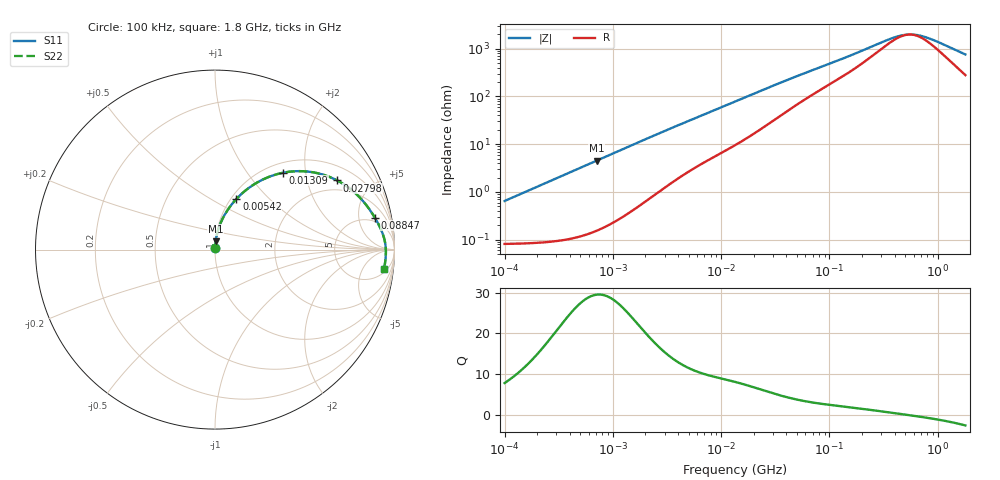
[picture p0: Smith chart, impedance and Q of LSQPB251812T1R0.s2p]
! LSQPB251812T1R0  S-PARAMETER MODEL  ( General Type )
! Model Generated by TAIYO YUDEN Corporation (http://www.ty-top.com)
! Version 3.0
! TAIYO YUDEN Control No. 110926NF18SB-HKC
! Copyright(c) 2007 TAIYO YUDEN CO.,LTD. All Rights Reserved.
! Product Description (link to TY-COMPAS)
! https://ds.yuden.co.jp/TYCOMPAS/or/detail?pn=LSQPB251812T1R0M&u=M
! Products Name : Inductors
! Characteristics :
!  Inductance : 1.0 uH , SRF(min) : 130 MHz , DC Resistance(max) : 0.104 Ohm
!  Rated Current : Saturation :1600 mA , Temp Rise : 1000 mA (40 degC)
!  Case Size : 2.5 x 1.8 / 0.098 x 0.071 [mm/inch] , Thickness : 1.2 / 0.048 [mm/inch]
!  (Conditions: Temperature = 25 degC , DC Bias Current/Voltage = 0A / 0V)
! External Node Assignments :
!  1  o---GGG---o  2
! GND o---------o GND
! Frequency Range : 0.1MHz  -  1800MHz  [ 402 STEP ]
# MHz S RI R 50
! Freq[MHz].  S11 Real  S11 Imag  S21 Real  S21 Imag  S12 Real  S12 Imag  S22 Real  S22 Imag
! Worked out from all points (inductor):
!   401 points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, 100 kHz to 1.8 GHz, reference 50 ohm
!   read as one part in series: L = 1.02 uH near 105 kHz
!   highest Q = 29.5 at 709.7 kHz (marker M1), where L = 1.02 uH
!   self-resonance near 546.1 MHz
!   S11 on the Smith chart (normalised r, x): 100 kHz: 1.00, +0.01; 5.42 MHz: 1.06, +0.66; 13.09 MHz: 1.18, +1.51; 27.98 MHz: 1.55, +3.08; 88.47 MHz: 4.01, +8.15; 1.8 GHz: 7, -14
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0.1  0.000855 0.0064  0.9991 -0.0064  0.9991 -0.0064  0.000855 0.0064
0.516129  0.00228 0.0329  0.9977 -0.0329  0.9977 -0.0329  0.00228 0.0329
0.709667  0.00359 0.0452  0.9964 -0.0452  0.9964 -0.0452  0.00359 0.0452
1.443982  0.0121 0.0905  0.9879 -0.0905  0.9879 -0.0905  0.0121 0.0905
2.66389  0.0365 0.16  0.9635 -0.16  0.9635 -0.16  0.0365 0.16
3.846706  0.0689 0.2183  0.9311 -0.2183  0.9311 -0.2183  0.0689 0.2183
5.420303  0.1193 0.2822  0.8807 -0.2822  0.8807 -0.2822  0.1193 0.2822
8.423854  0.2241 0.3675  0.7759 -0.3675  0.7759 -0.3675  0.2241 0.3675
13.09176  0.3803 0.4284  0.6197 -0.4284  0.6197 -0.4284  0.3803 0.4284
13.41641  0.3902 0.4303  0.6098 -0.4303  0.6098 -0.4303  0.3902 0.4303
18.90474  0.533 0.4327  0.467 -0.4327  0.467 -0.4327  0.533 0.4327
27.97575  0.6805 0.3855  0.3195 -0.3855  0.3195 -0.3855  0.6805 0.3855
42.42587  0.7912 0.3056  0.2088 -0.3056  0.2088 -0.3056  0.7912 0.3056
69.24595  0.8666 0.2155  0.1334 -0.2155  0.1334 -0.2155  0.8666 0.2155
88.46596  0.8906 0.178  0.1094 -0.178  0.1094 -0.178  0.8906 0.178
159.2548  0.9278 0.1053  0.0722 -0.1053  0.0722 -0.1053  0.9278 0.1053
357.3983  0.9489 0.0319  0.0511 -0.0319  0.0511 -0.0319  0.9489 0.0319
491.4156  0.9515 0.00781  0.0485 -0.00781  0.0485 -0.00781  0.9515 0.00781
569.2172  0.952 -0.00307  0.048 0.00307  0.048 0.00307  0.952 -0.00307
659.3364  0.9522 -0.0141  0.0478 0.0141  0.0478 0.0141  0.9522 -0.0141
884.6373  0.9514 -0.0373  0.0486 0.0373  0.0486 0.0373  0.9514 -0.0373
1800  0.9404 -0.1104  0.0596 0.1104  0.0596 0.1104  0.9404 -0.1104
